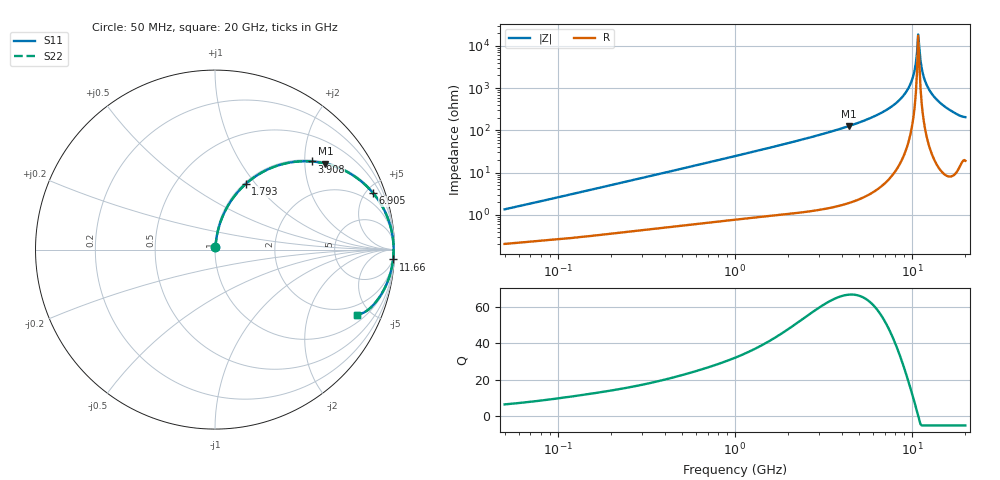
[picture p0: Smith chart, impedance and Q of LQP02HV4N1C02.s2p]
!Murata Part Number: LQP02HV4N1C02
!These Parameters are Measured in Series Mode Connection
!  o--[Z]--o
!Port1  Port2
!  o-------o
!Freq. Start=50[MHz] Stop=20[GHz], 401[Steps]
# Hz S RI R 50
!Freq.(Hz) S11(Real) S11(Imag) S21(Real) S21(Imag) S12(Real) S12(Imag) S22(Real) S22(Imag)
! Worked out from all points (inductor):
!   401 points, 50 MHz to 20 GHz, reference 50 ohm
!   read as one part in series: L = 4.19 nH near 51.52 MHz
!   highest Q = 66.6 at 4.406 GHz (marker M1), where L = 4.59 nH
!   self-resonance near 10.82 GHz
!   S11 on the Smith chart (normalised r, x): 50 MHz: 1.00, +0.03; 1.793 GHz: 1.02, +0.89; 3.908 GHz: 1.03, +2.16; 6.905 GHz: 1.10, +5.58; 11.66 GHz: 4, -36; 20 GHz: 1.38, -4.11
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5e7  0.00222 0.0133  0.9978 -0.0133  0.9978 -0.0133  0.00222 0.0133
1.364002e8  0.0042 0.0347  0.9958 -0.0347  0.9958 -0.0347  0.0042 0.0347
3.721004e8  0.0132 0.0909  0.9868 -0.0909  0.9868 -0.0909  0.0132 0.0909
1e9  0.0634 0.2286  0.9366 -0.2286  0.9366 -0.2286  0.0634 0.2286
1.793498e9  0.1716 0.366  0.8284 -0.366  0.8284 -0.366  0.1716 0.366
2.728004e9  0.3333 0.4627  0.6667 -0.4627  0.6667 -0.4627  0.3333 0.4627
3.908127e9  0.5386 0.4909  0.4614 -0.4909  0.4614 -0.4909  0.5386 0.4909
4.405649e9  0.6156 0.479  0.3844 -0.479  0.3844 -0.479  0.6156 0.479
6.905011e9  0.8815 0.3139  0.1185 -0.3139  0.1185 -0.3139  0.8815 0.3139
7.442007e9  0.9146 0.2692  0.0854 -0.2692  0.0854 -0.2692  0.9146 0.2692
8.644534e9  0.9649 0.1689  0.0351 -0.1689  0.0351 -0.1689  0.9649 0.1689
9.600142e9  0.9861 0.0925  0.0139 -0.0925  0.0139 -0.0925  0.9861 0.0925
1.019291e10  0.9927 0.0475  0.00731 -0.0475  0.00731 -0.0475  0.9927 0.0475
1.050288e10  0.9944 0.0248  0.0056 -0.0248  0.0056 -0.0248  0.9944 0.0248
1.082228e10  0.995 0.00194  0.00495 -0.00194  0.00495 -0.00194  0.995 0.00194
1.115139e10  0.9946 -0.0209  0.00536 0.0209  0.00536 0.0209  0.9946 -0.0209
1.149051e10  0.9932 -0.0437  0.00684 0.0437  0.00684 0.0437  0.9932 -0.0437
1.166392e10  0.992 -0.0551  0.00798 0.0551  0.00798 0.0551  0.992 -0.0551
1.257102e10  0.9823 -0.1115  0.0177 0.1115  0.0177 0.1115  0.9823 -0.1115
1.417136e10  0.9531 -0.1985  0.0469 0.1985  0.0469 0.1985  0.9531 -0.1985
1.696185e10  0.8763 -0.3143  0.1237 0.3143  0.1237 0.3143  0.8763 -0.3143
2e10  0.7885 -0.3645  0.2115 0.3645  0.2115 0.3645  0.7885 -0.3645
